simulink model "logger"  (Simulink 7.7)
settings: Solver=FixedStepDiscrete  SolverMode=SingleTasking  StartTime=0.0  StopTime=60.0  RelTol=1e-3  AbsTol=1e-6
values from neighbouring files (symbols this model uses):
  h = 0.05    [initlab3.m]
libraries: newlab3_lib x2

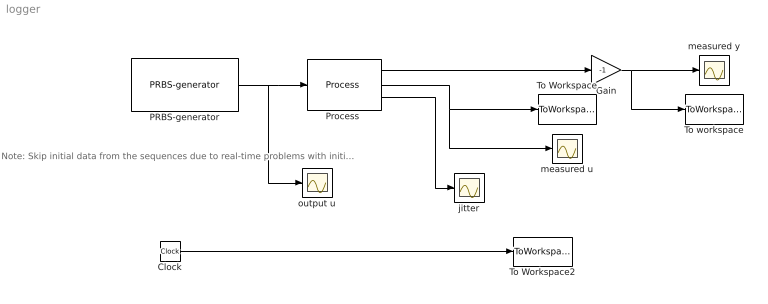
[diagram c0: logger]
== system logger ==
  note: Note: Skip initial data from the sequences due to real-time problems with initialization (see the jitter-plot)
  Clock : Clock
  Gain : Gain  Gain=-1
  PRBS-generator : newlab3_lib/PRBS-generator  SystemSampleTime=-1  h=h  N=10  Amp=0.5  offset=0.8  seed=0
  "Process " : newlab3_lib/Process   SystemSampleTime=-1  AOu=0  AIy=0  AIu=1  h=h
  To Workspace : ToWorkspace  VariableName=u  SampleTime=h  SaveFormat=Array
  To Workspace2 : ToWorkspace  VariableName=time  SampleTime=-1  SaveFormat=Array
  To workspace : ToWorkspace  VariableName=y  SampleTime=h  SaveFormat=Array
  jitter : Scope
  measured u : Scope
  measured y : Scope
  output u : Scope
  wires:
  "Process "/3 -> jitter/1
  Clock/1 -> To Workspace2/1
  "Process "/2 -> measured u/1, To Workspace/1
  PRBS-generator/1 -> "Process "/1, output u/1
  "Process "/1 -> Gain/1
  Gain/1 -> measured y/1, To workspace/1
